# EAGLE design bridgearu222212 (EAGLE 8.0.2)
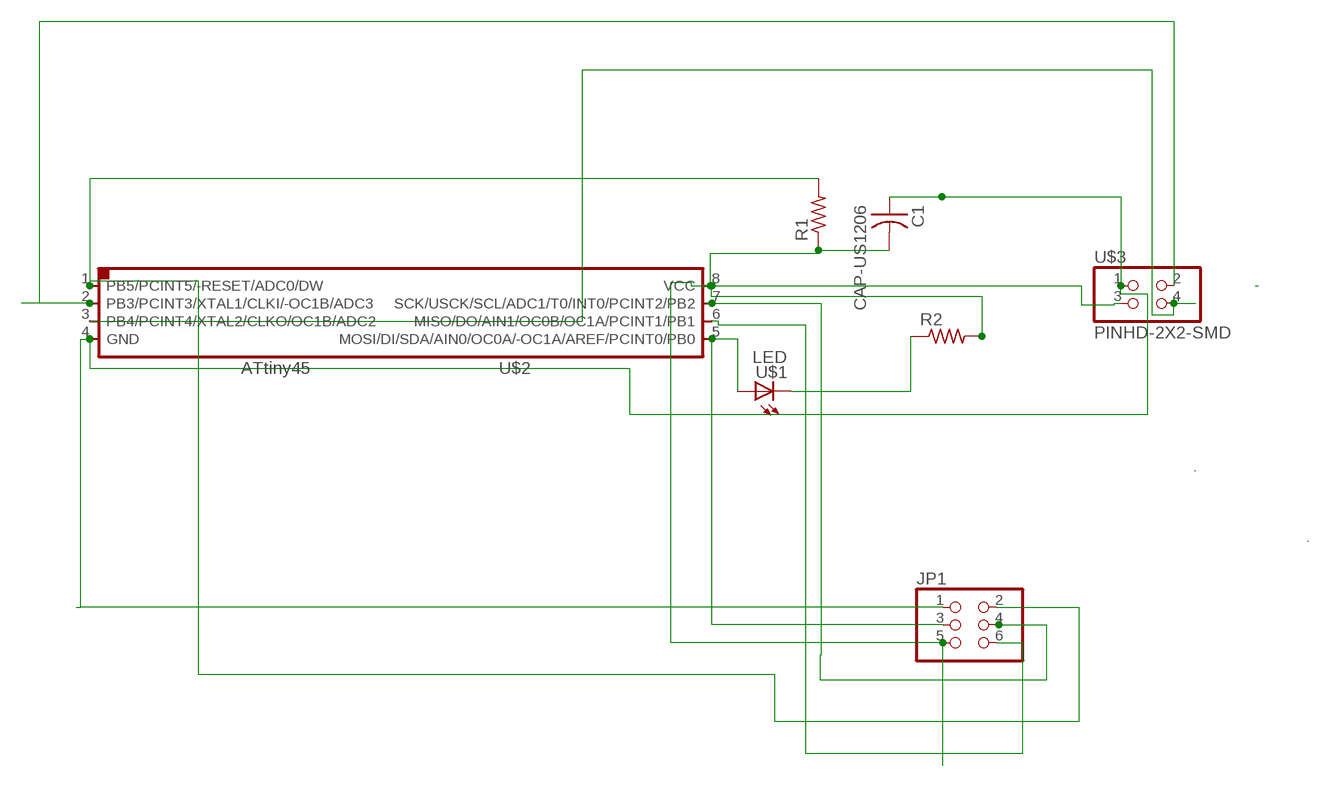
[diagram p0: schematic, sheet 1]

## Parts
C1  CAP-US1206  [C1206]
JP1  PINHD-2X3-SMD  [2X03SMD]
R1  RES-US1206  [R1206]
R2  RES-US1206  [R1206]
U$1  LED  [LED1206]
U$2  ATTINY45SI  [SOIC8]
U$3  PINHD-2X2-SMD  [2X02SMD]

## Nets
N$4: JP1.2 R1.2 U$2.1(PB5/PCINT5/-RESET/ADC0/DW)
N$6: JP1.3 U$1.1(A) U$2.5(MOSI/DI/SDA/AIN0/OC0A/-OC1A/AREF/PCINT0/PB0)
N$7: R2.1 U$1.2(C)
N$8: U$2.3(PB4/PCINT4/XTAL2/CLKO/OC1B/ADC2) U$3.4
N$13: C1.2 JP1.5 R1.1 R2.2 U$2.8(VCC) U$3.3
N$15: JP1.4 U$2.7(SCK/USCK/SCL/ADC1/T0/INT0/PCINT2/PB2)
N$17: JP1.6 U$2.6(MISO/DO/AIN1/OC0B/OC1A/PCINT1/PB1)
N$18: C1.1 JP1.1 U$2.4(GND) U$3.1
N$19: U$2.2(PB3/PCINT3/XTAL1/CLKI/-OC1B/ADC3) U$3.2

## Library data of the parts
C1 = fab:CAP-US
JP1 = fab:PINHD-2X3-SMD: PIN HEADER
R1 R2 = fab:RES-US: Resistor (US Symbol)
U$1 = fab:LED: LED
U$2 = fab:ATTINY45
U$3 = fab:PINHD-2X2-SMD

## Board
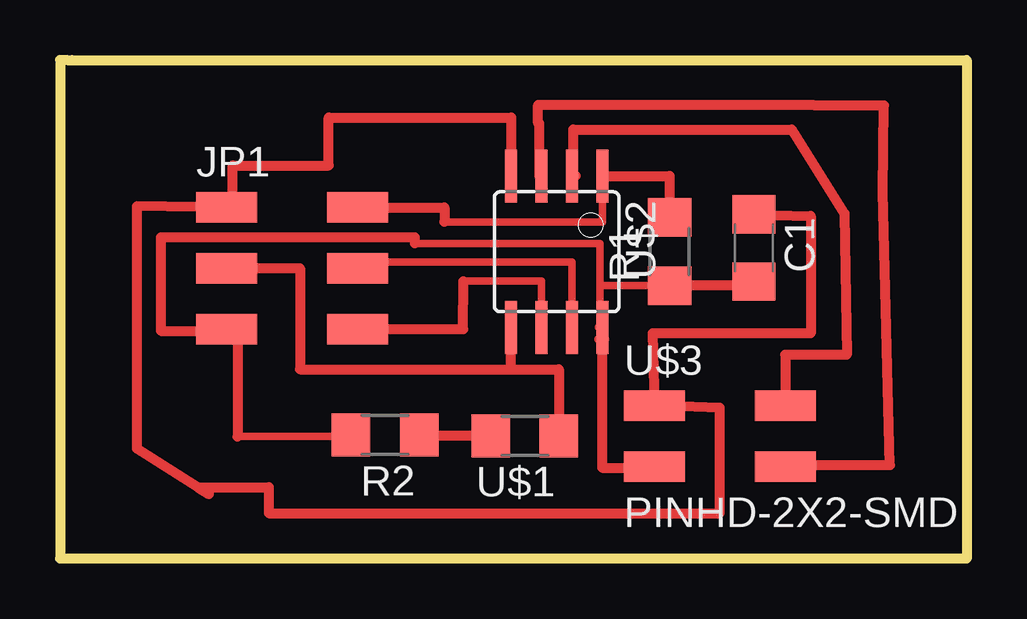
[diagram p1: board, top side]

Size 37.8 x 20.8 mm. Coordinates in mm from the lower left corner, seen from the top.
Outline: 0.3,20.8 0.5,20.8 37.8,20.8 37.8,0 0,0 0,20.8 0.3,20.8
Copper layers (1*16): Top 0.035mm / dielectric 1.5mm / Bottom 0.035mm
Design rules "default": minimum track width 10mil, minimum drill 24mil, track to track 8mil, track to pad 8mil, pad to pad 8mil, via to via 8mil, smd to smd 8mil, copper to edge 40mil, drill to drill 8mil, minimum pad ring 10mil, minimum via ring 8mil, stop-mask expansion 4mil, vias tented up to drill 0mil, thermal gap 10mil

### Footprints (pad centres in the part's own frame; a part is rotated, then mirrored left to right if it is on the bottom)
C1206 = smd 1.6 x 1.8: 1 -1.4,0; 2 1.4,0
2X03SMD = smd 2.54 x 1.27: 1 -2.54,2.54; 2 2.92,2.54; 3 -2.54,0; 4 2.92,0; 5 -2.54,-2.54; 6 2.92,-2.54
R1206 = smd 1.6 x 1.803: 1 -1.422,0; 2 1.422,0
LED1206 = smd 1.6 x 1.803: 1 -1.422,0; 2 1.422,0
SOIC8 = smd 0.5 x 2.2: 1 -1.905,-3.154; 2 -0.645,-3.154; 3 0.625,-3.154; 4 1.895,-3.154; 5 1.905,3.154; 6 0.635,3.154; 7 -0.635,3.154; 8 -1.905,3.154
2X02SMD = smd 2.54 x 1.27: 1 -2.54,1.27; 2 2.92,1.27; 3 -2.54,-1.27; 4 2.92,-1.27

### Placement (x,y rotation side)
C1  28.93,12.96 270 top
JP1  9.48,12.11 0 top
R1  25.41,12.81 90 top
R2  13.55,5.16 180 top
U$1  19.37,5.13 180 top
U$2  20.71,12.8 180 top
U$3  27.32,5.11 0 top

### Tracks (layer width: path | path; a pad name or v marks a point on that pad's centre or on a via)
N$4
  Top 0.305: 16.03,14.05 22.61,14.05 U$2.1
  Top 0.406: JP1.2 16.03,14.65 16.03,14.05 | U$2.1 25.41,15.96 R1.2
N$6
  Top 0.406: 8.13,12.11 JP1.3 10,12.11 10,7.9 18.8,7.9 | 18.8,7.9 U$2.5 | 18.8,7.9 20.8,7.9 U$1.1
N$7
  Top 0.406: U$1.2 14.98,5.13 R2.1
N$8
  Top 0.305: 31.45,18.9 31.4,18.92
  Top 0.406: U$2.3 19.99,15.96 19.99,18.16 19.94,18.16 19.94,18.92 31.4,18.92 | 30.23,3.8 U$3.4 30.23,3.9 34.6,3.9 34.3,15.3 34.35,18.9 31.45,18.9
N$13
  Top 0.305: 14.8,13.15 22.5,13.15 22.5,11.5 22.5,11.39 | 22.5,11.39 22.5,9.14 | R1.1 22.5,11.39 | 7.4,5.1 12.13,5.1 R2.2
  Top 0.406: 22.61,9.14 22.5,9.14 22.48,9.14 | 22.68,9.14 22.61,9.14 | 22.61,9.14 U$2.8 | R1.1 28.93,11.39 C1.2 | U$2.8 22.5,9.65 | 14.8,13.15 14.8,13.4 4.2,13.4 4.2,9.5 6.94,9.5 JP1.5 7.4,9.57 7.4,5.1 | R2.2 12.13,5.1 | U$2.8 22.6,3.8 24.78,3.8 U$3.3
N$15
  Top 0.305: U$2.7 21.34,12.36 12.4,12.36
  Top 0.406: 12.4,12.36 JP1.4
N$17
  Top 0.305: 16.81,11.58 20.07,11.58 U$2.6
  Top 0.406: JP1.6 16.81,9.57 16.81,11.58
N$18
  Top 0.406: 5.93,14.65 JP1.1 | U$2.4 18.86,15.96 | U$3.1 24.9,6.38 | JP1.1 7.36,14.65 | 18.81,17.1 U$2.4 | JP1.1 3.2,14.7 3.2,4.6 5.75,2.98 | 5.75,2.98 6.2,2.7 | U$3.1 27.5,6.3 27.5,1.9 8.7,1.9 8.7,2.98 5.75,2.98 | C1.1 31.3,14.3 31.3,9.4 24.7,9.4 U$3.1 | JP1.1 7.2,14.65 7.2,16.4 11.2,16.4 11.2,18.4 18.81,18.4 U$2.4
N$19
  Top 0.406: 21.5,15.96 U$2.2 21.4,15.96 21.4,17.9 30.5,17.9 32.7,14.4 32.8,8.5 30.23,8.5 U$3.2 30.23,6.4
